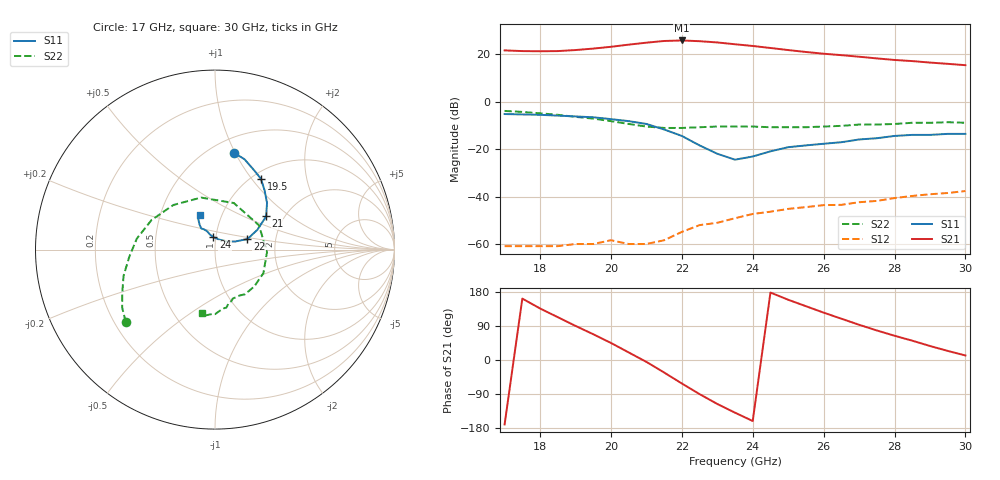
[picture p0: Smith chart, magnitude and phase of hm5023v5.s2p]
! HMMC-5023
! S-PARAMETERS  at  Vdd = 5V.  LAST UPDATED 02-24-97
#  GHZ  S  MA  R 50
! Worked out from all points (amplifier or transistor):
!   27 points, 17 GHz to 30 GHz, reference 50 ohm
!   highest |S21| = 25.8 dB at 22 GHz (marker M1)
!   |S21| within 3 dB of that: 19.79 GHz to 24.4 GHz (4.611 GHz wide, 20.9 % of centre)
!   unconditionally stable (mu >= 1): start of sweep to end of sweep
!   at 19 GHz: K = 23.56, MAG = 24.2 dB, |S12| = -60.0 dB
!   at 23.5 GHz: K = 7.97, MAG = 24.7 dB, |S12| = -49.1 dB
!   at 30 GHz: K = 5.40, MAG = 16.2 dB, |S12| = -37.7 dB
!   S11 on the Smith chart (normalised r, x): 17 GHz: 0.64, +0.99; 19.5 GHz: 1.10, +1.11; 21 GHz: 1.62, +0.68; 22 GHz: 1.43, +0.17; 24 GHz: 0.97, +0.14; 30 GHz: 0.79, +0.32
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17  0.55 79.0  12.1 -170.0  0.0009 173.0  0.64 -141.0
17.5  0.54 76.0  11.7 162.0  0.0009 164.0  0.61 -148.0
18  0.53 72.0  11.6 136.0  0.0009 162.0  0.57 -155.0
18.5  0.51 68.0  11.7 113.0  0.0009 143.0  0.53 -164.0
19  0.49 63.0  12.3 90.0  0.001 139.0  0.48 -175.0
19.5  0.47 57.0  13.2 68.0  0.001 110.0  0.44 172.0
20  0.43 50.0  14.4 45.0  0.0012 80.0  0.39 155.0
20.5  0.39 42.0  16 20.0  0.001 50.0  0.34 133.0
21  0.34 33.0  17.6 -5.0  0.001 28.0  0.3 105.0
21.5  0.26 25.0  19.1 -33.0  0.0012 -14.0  0.28 68.0
22  0.19 18.0  19.6 -62.0  0.0018 -70.0  0.28 29.0
22.5  0.12 22.0  18.9 -90.0  0.0025 -93.0  0.29 -3.0
23  0.08 35.0  17.8 -116.0  0.0028 -114.0  0.3 -26.0
23.5  0.06 69.0  16.3 -139.0  0.0035 -136.0  0.3 -43.0
24  0.07 97.0  15 -161.0  0.0043 -154.0  0.3 -56.0
24.5  0.09 109.0  13.6 178.0  0.0048 -166.0  0.29 -62.0
25  0.11 113.0  12.3 159.0  0.0055 177.0  0.29 -67.0
26  0.13 119.0  10.3 125.0  0.0066 151.0  0.3 -72.0
27  0.16 122.0  8.9 93.0  0.0076 136.0  0.33 -79.0
28  0.19 119.0  7.6 64.0  0.0093 114.0  0.34 -85.0
29  0.2 116.0  6.7 37.0  0.0112 93.0  0.36 -93.0
30  0.21 113.0  5.9 12.0  0.0131 76.0  0.36 -102.0
